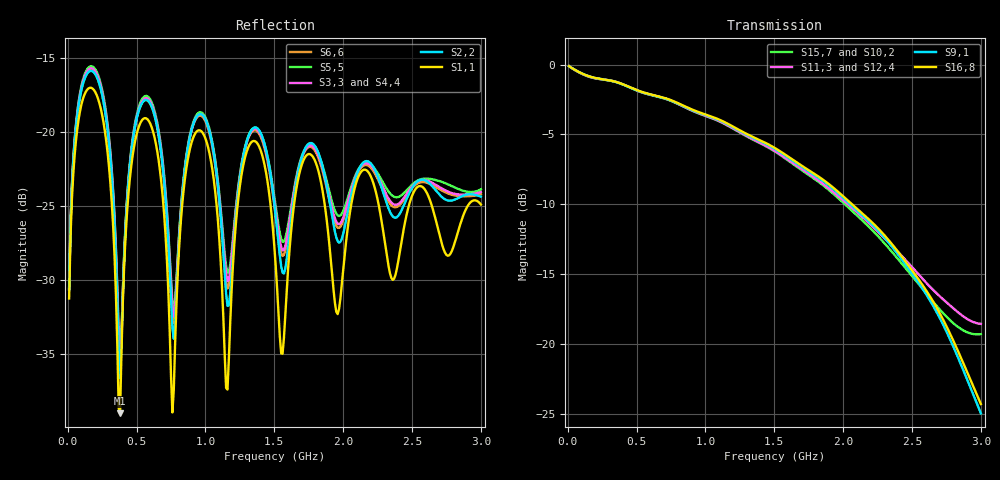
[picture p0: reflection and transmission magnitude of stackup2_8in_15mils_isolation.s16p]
! Touchstone file from project
# GHZ S RI R 50.000000
! Modal data exported
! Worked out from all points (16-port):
!   300 points, 10 MHz to 3 GHz, reference 50 ohm
!   strongest paths, dB at 10 MHz, 760 MHz, 1.51 GHz, 2.26 GHz, 3 GHz:
!     S16,8: -0.1, -2.6, -6.0, -11.8, -24.3
!     S9,1: -0.1, -2.6, -6.1, -11.9, -24.9
!     S11,3: -0.1, -2.6, -6.2, -12.0, -18.5
!     S12,4: -0.1, -2.6, -6.2, -12.1, -18.8
!     S15,7: -0.1, -2.6, -6.3, -12.3, -19.3
!     S10,2: -0.1, -2.6, -6.3, -12.4, -19.2
!   lowest |S11| = -39.0 dB at 380 MHz (marker M1), VSWR 1.02, Z = 51.1 + j0.21 ohm
!   |S11| at or under -10 dB: start of sweep to end of sweep
